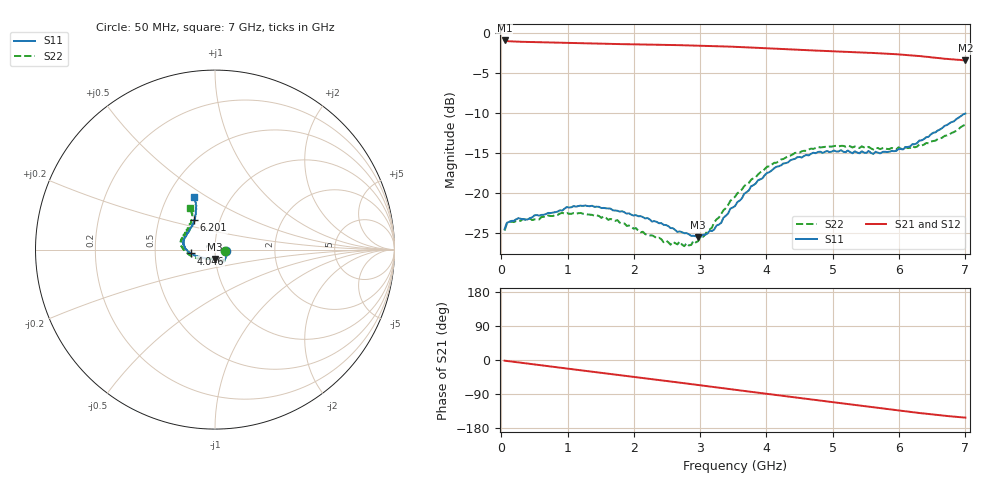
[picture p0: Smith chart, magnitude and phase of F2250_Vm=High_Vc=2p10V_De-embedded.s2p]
! Integrated Device Technology
! Corporate Headquarters
! 6024 Silver Creek Valley Road
! San Jose, CA 95138  USA
! Phone:  1-408-284-8200
! Toll Free:  1-800-223-1366
! Webpage:  http://www.idt.com/
! Timing and RF Division
! 515 Groton Road, Suite 102
! Westford, MA 01886-6024
! Device:  F2250
! Description: Voltage Variable RF Attenuator
! Frequency:  50.0 -  6000.00 MHz
! Package:  3x3 mm Thin QFN Plastic Package: 16 pin
! Ports:  2 RF, 3 DC
!  Pin  1  = GND
!  Pin  2  = NC
!  Pin  3  = RF1  = Port 1
!  Pin  4  = NC
!  Pin  5  = GND
!  Pin  6  = GND
!  Pin  7  = GND
!  Pin  8  = GND
!  Pin  9  = NC
!  Pin 10  = RF2  = Port 2
!  Pin 11  = NC
!  Pin 12  = GND
!  Pin 13  = GND
!  Pin 14  = VCNTRL
!  Pin 15  = VDD
!  Pin 16  = VMODE
! Vcntrl:  2.100 Volts
! Vmode:  +3.300 Volts
! Vdd:  +3.30  Volts
! Current:  1.318 mA
! Data:  The device was measured on a the F2250 evaluation board which has
!  individual transmission lines to the RF pins.  Data was collected
!  using a calibrated network analyzer.  The evaluation board was
!  de-embedded using a TRL calibration technique.
!  The reference plane is the edge of the package pin.
! Misc:  SN 10
!  Action Tracker AT0258
! Date Measured:  2014-11-26
! Date:  2015-10-15  MJV
! Note:
!  Integrated Device Technology supplies this data as a sample of measured
!  data at the package pin for this product.  Your particular data for this
!  product may vary.
!  Data was taken at 25 degrees C.
!  Integrated Device Technology reserves the right to change this data at anytime.
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# GHz S dB R 50
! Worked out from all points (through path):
!   201 points, 50 MHz to 7 GHz, reference 50 ohm
!   highest |S21| = -0.96 dB at 50 MHz (marker M1); lowest = -3.4 dB at 7 GHz (marker M2)
!   group delay of S21, straight-line fit = 61.1 ps
!   lowest |S11| = -25.5 dB at 2.969 GHz (marker M3), VSWR 1.11, Z = 49.6 - j5.27 ohm
!   |S11| at or under -10 dB: start of sweep to end of sweep
!   |S22| runs from -26.6 to -11.5 dB; largest |S21 - S12| = 0.0019
!   S11 on the Smith chart (normalised r, x): 50 MHz: 1.13, -0.02; 4.046 GHz: 0.76, -0.03; 6.201 GHz: 0.75, +0.26; 7 GHz: 0.68, +0.44
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0.05  -24.48 -9.3  -0.96 -1.8  -0.96 -1.8  -24.67 -9.9
0.08475  -23.70 -8.6  -1.04 -2.5  -1.03 -2.5  -23.77 -8.8
0.1195  -23.59 -9.2  -1.07 -3.3  -1.06 -3.2  -23.58 -8.3
0.91875  -22.17 -46.4  -1.25 -21.0  -1.25 -21.1  -22.45 -48.9
1.2315  -21.60 -54.2  -1.32 -27.9  -1.32 -27.9  -22.56 -59.3
1.75275  -22.20 -61.1  -1.41 -39.1  -1.41 -39.1  -23.38 -66.6
2.37825  -23.75 -61.3  -1.50 -52.8  -1.50 -52.8  -25.56 -68.7
2.552  -24.35 -65.8  -1.53 -56.6  -1.53 -56.6  -26.43 -75.2
2.691  -24.77 -72.9  -1.55 -59.7  -1.55 -59.7  -26.04 -82.4
2.7605  -25.00 -74.9  -1.56 -61.3  -1.57 -61.3  -26.62 -86.7
2.969  -25.52 -91.0  -1.60 -65.9  -1.60 -66.0  -25.99 -104.5
3.21225  -24.54 -120.2  -1.66 -71.4  -1.66 -71.5  -23.64 -128.3
3.525  -21.63 -147.2  -1.76 -78.5  -1.76 -78.5  -20.46 -147.0
3.76825  -19.15 -160.7  -1.85 -84.0  -1.85 -84.0  -18.33 -158.3
4.04625  -17.38 -170.8  -1.96 -90.2  -1.96 -90.2  -16.67 -168.8
4.4285  -15.74 178.6  -2.11 -98.6  -2.11 -98.6  -14.99 179.6
4.7065  -14.96 171.4  -2.20 -104.8  -2.21 -104.8  -14.49 173.7
5.054  -14.81 163.2  -2.34 -112.4  -2.33 -112.5  -14.10 166.6
5.85325  -14.84 137.0  -2.63 -129.9  -2.63 -130.1  -14.50 147.6
6.20075  -13.89 125.1  -2.84 -137.7  -2.84 -137.7  -14.11 138.6
6.54825  -12.42 116.8  -3.11 -144.7  -3.11 -144.8  -13.46 127.2
7  -10.09 111.8  -3.44 -152.0  -3.45 -152.1  -11.46 120.9
